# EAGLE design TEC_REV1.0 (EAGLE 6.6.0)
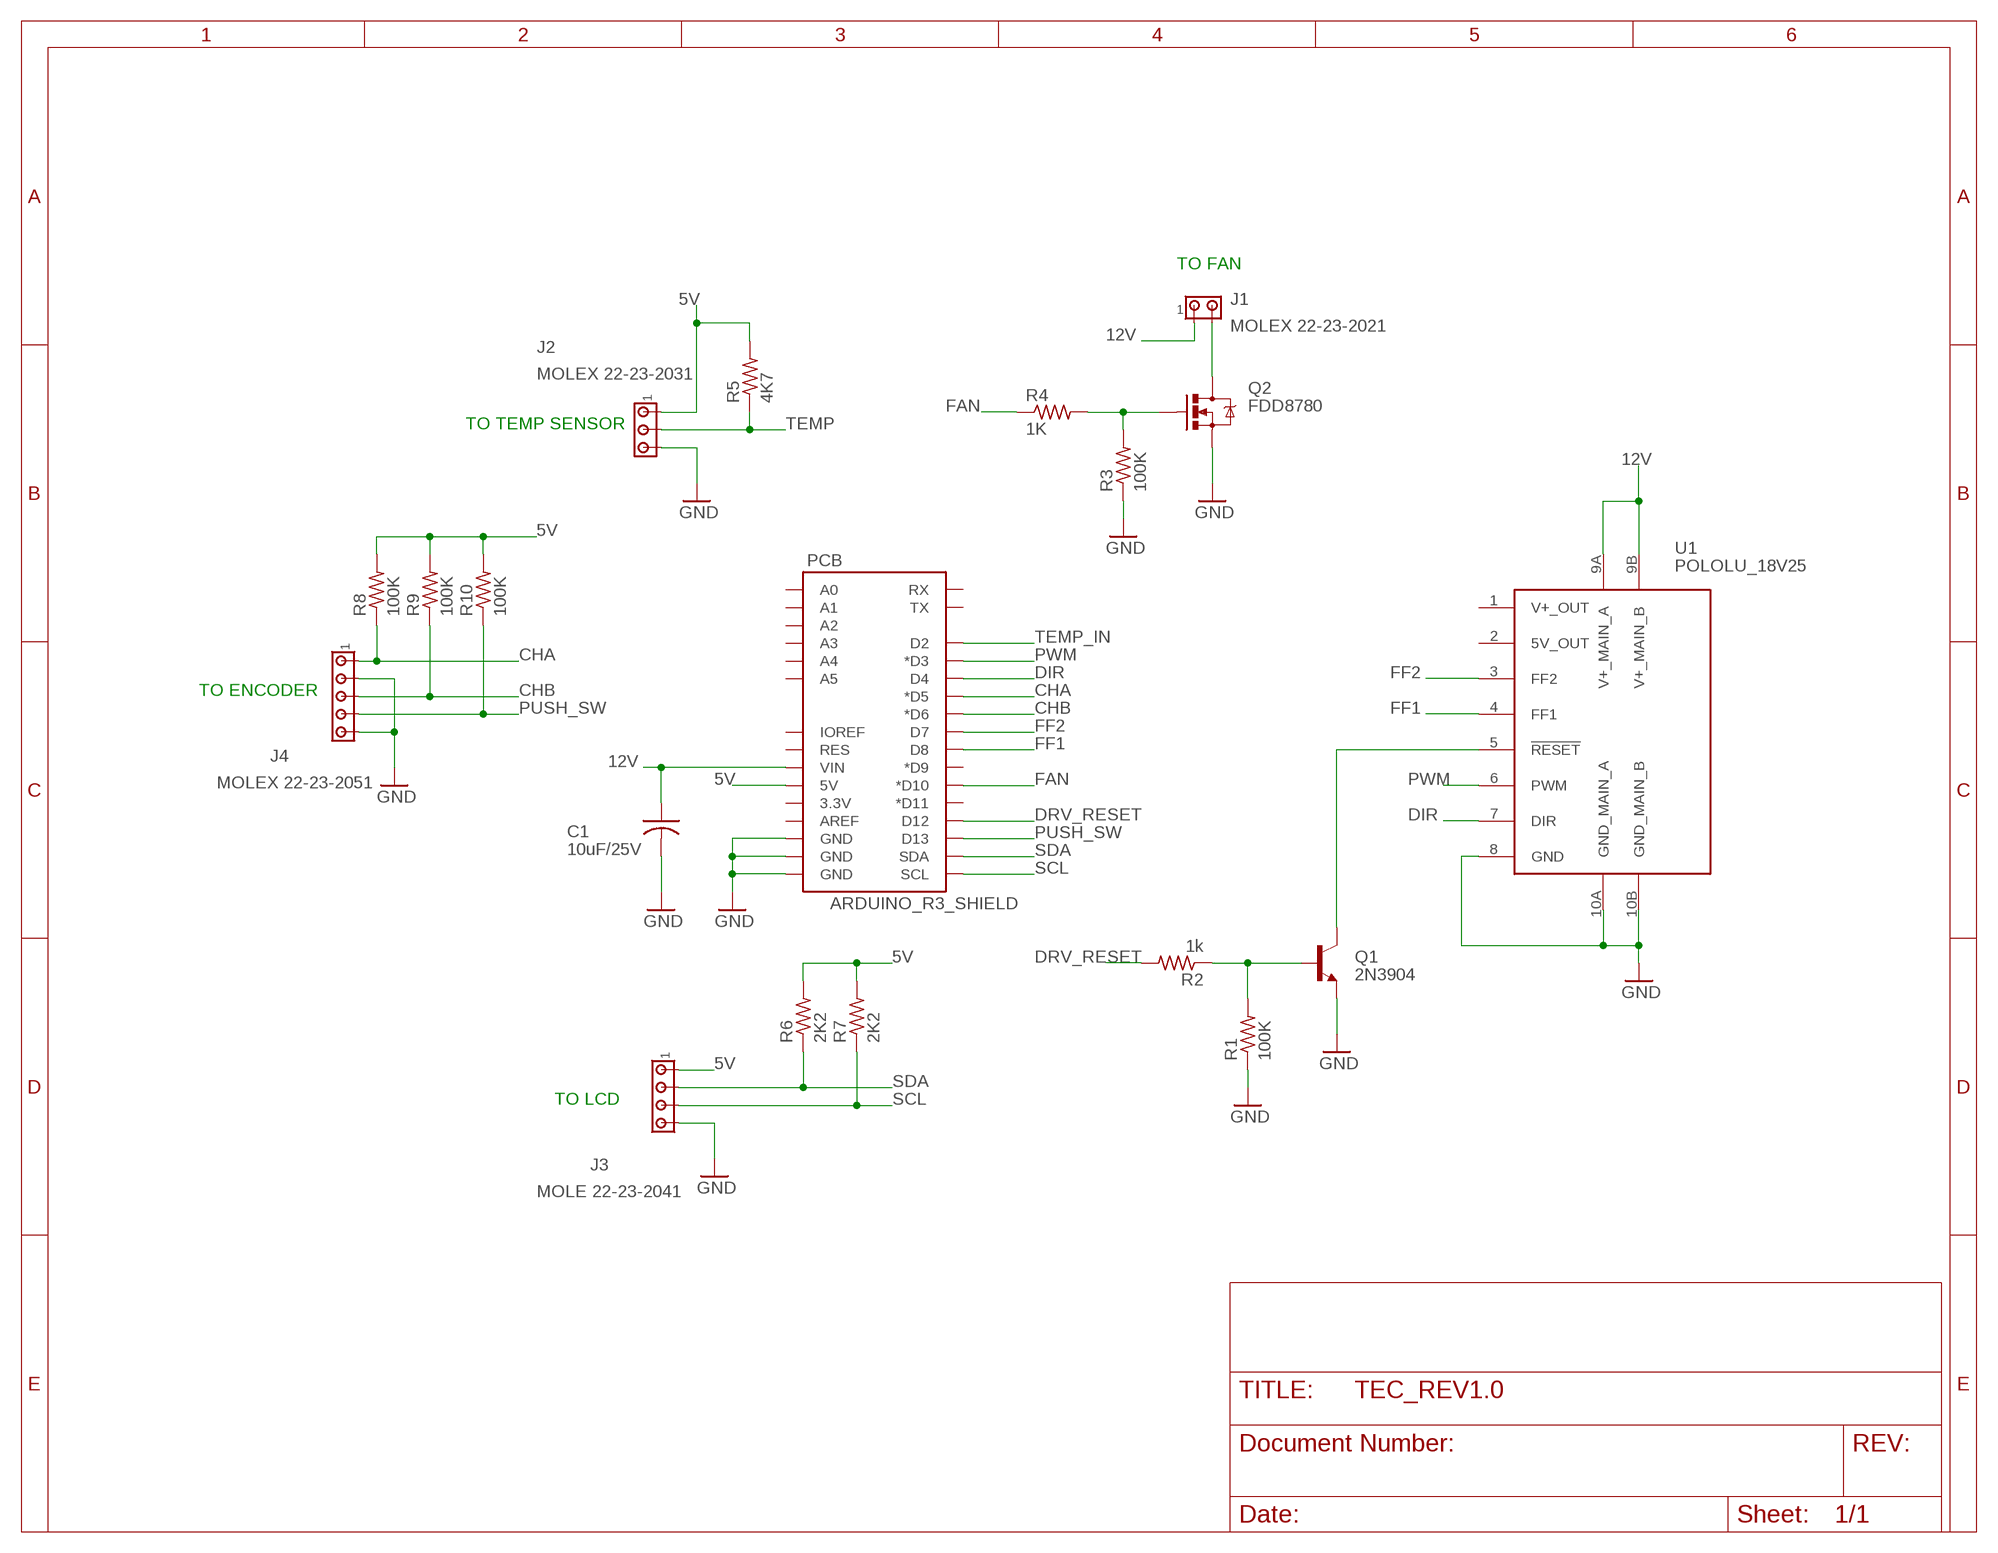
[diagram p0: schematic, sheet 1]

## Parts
C1  10uF/25V  C-USC0603  [C0603]
J1  MOLEX 22-23-2021  MTA02-100  [10X02MTA]
J2  MOLEX 22-23-2031  MTA03-100  [10X03MTA]
J3  MOLE 22-23-2041  MTA04-100  [10X04MTA]
J4  MOLEX 22-23-2051  MTA05-100  [10X05MTA]
PCB  ARDUINO_R3_SHIELD  [UNO_R3_SHIELD]
Q1  2N3904  TRANSISTOR_NPNSOT23  [SOT23]
Q2  FDD8780  MOSFET-NCHANNELFDD8780  [DPAK]
R1  100K  R-US_R0603  [R0603]
R2  1k  R-US_R0603  [R0603]
R3  100K  R-US_R0603  [R0603]
R4  1K  R-US_R0603  [R0603]
R5  4K7  R-US_R0603  [R0603]
R6  2K2  R-US_R0603  [R0603]
R7  2K2  R-US_R0603  [R0603]
R8  100K  R-US_R0603  [R0603]
R9  100K  R-US_R0603  [R0603]
R10  100K  R-US_R0603  [R0603]
U1  POLOLU_18V25  [POLOLU_18V25]

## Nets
5V: J2.1 J3.1 PCB.5V R5.2 R6.2 R7.2 R8.2 R9.2 R10.2
12V: C1.1 J1.1 PCB.VIN U1.9A(V+_MAIN_A) U1.9B(V+_MAIN_B)
CHA: J4.1 PCB.D5(*D5) R8.1
CHB: J4.3 PCB.D6(*D6) R9.1
DIR: PCB.D4 U1.7(DIR)
DRV_RESET: PCB.D12 R2.2
FAN: PCB.D10(*D10) R4.1
FF1: PCB.D8 U1.4(FF1)
FF2: PCB.D7 U1.3(FF2)
GND: C1.2 J2.3 J3.4 J4.2 J4.5 PCB.GND@0(GND) PCB.GND@1(GND) PCB.GND@2(GND) Q1.2(E) Q2.3(S) R1.1 R3.1 U1.8(GND) U1.10A(GND_MAIN_A) U1.10B(GND_MAIN_B)
N$2: Q1.3(C) U1.5(!RESET)
N$3: J1.2 Q2.4(D)
N$5: Q2.1(G) R3.2 R4.2
N$6: Q1.1(B) R1.2 R2.1
PUSH_SW: J4.4 PCB.D13 R10.1
PWM: PCB.D3(*D3) U1.6(PWM)
SCL: J3.3 PCB.SCL R7.1
SDA: J3.2 PCB.SDA R6.1
TEMP: J2.2 R5.1
TEMP_IN: PCB.D2
Unconnected: PCB.3.3V PCB.A0 PCB.A1 PCB.A2 PCB.A3 PCB.A4 PCB.A5 PCB.AREF PCB.D9(*D9) PCB.D11(*D11) PCB.IOREF PCB.RES PCB.RX PCB.TX U1.1(V+_OUT) U1.2(5V_OUT)

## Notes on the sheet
- TO FAN
- TO TEMP SENSOR
- TO ENCODER
- TO LCD

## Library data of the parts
C1 = rcl:C-US: CAPACITOR, American symbol
J1 = con-amp:MTA02-100: AMP connector
J2 = con-amp:MTA03-100: AMP connector
J3 = con-amp:MTA04-100: AMP connector
J4 = con-amp:MTA05-100: AMP connector
PCB = SparkFun-Boards:ARDUINO_R3_SHIELD: Shield form compatible with the Arduino Uno R3.
Q1 = SparkFun-DiscreteSemi:TRANSISTOR_NPN: Generic NPN BJT MMBT2222A - TRANS-08049 (SOT-23, 1A 40V) MPSA42 - TRANS-09116 (SOT-23, 500mA 300V) MMBT5088LT1G - TRANS-11160 (SOT-23, 50 mA 30V)
Q2 = SparkFun-DiscreteSemi:MOSFET-NCHANNEL: Common NMOSFET Parts MFG P/NStore IDProd ID FDD8780TRANS-09984 SI7820DNTRANS-11055 FDS6630AIC-08089 2N7002PWTRANS-11151 FQP30N06L COM-10213TRANS-10060 BSS123LT1GTRANS-08345 BSS138TRANS-00830 BS170 2N7000; PROD_ID: TRANS-09984
R1-R10 = rcl:R-US_: RESISTOR, American symbol
U1 = Dartronix:POLOLU_18V25

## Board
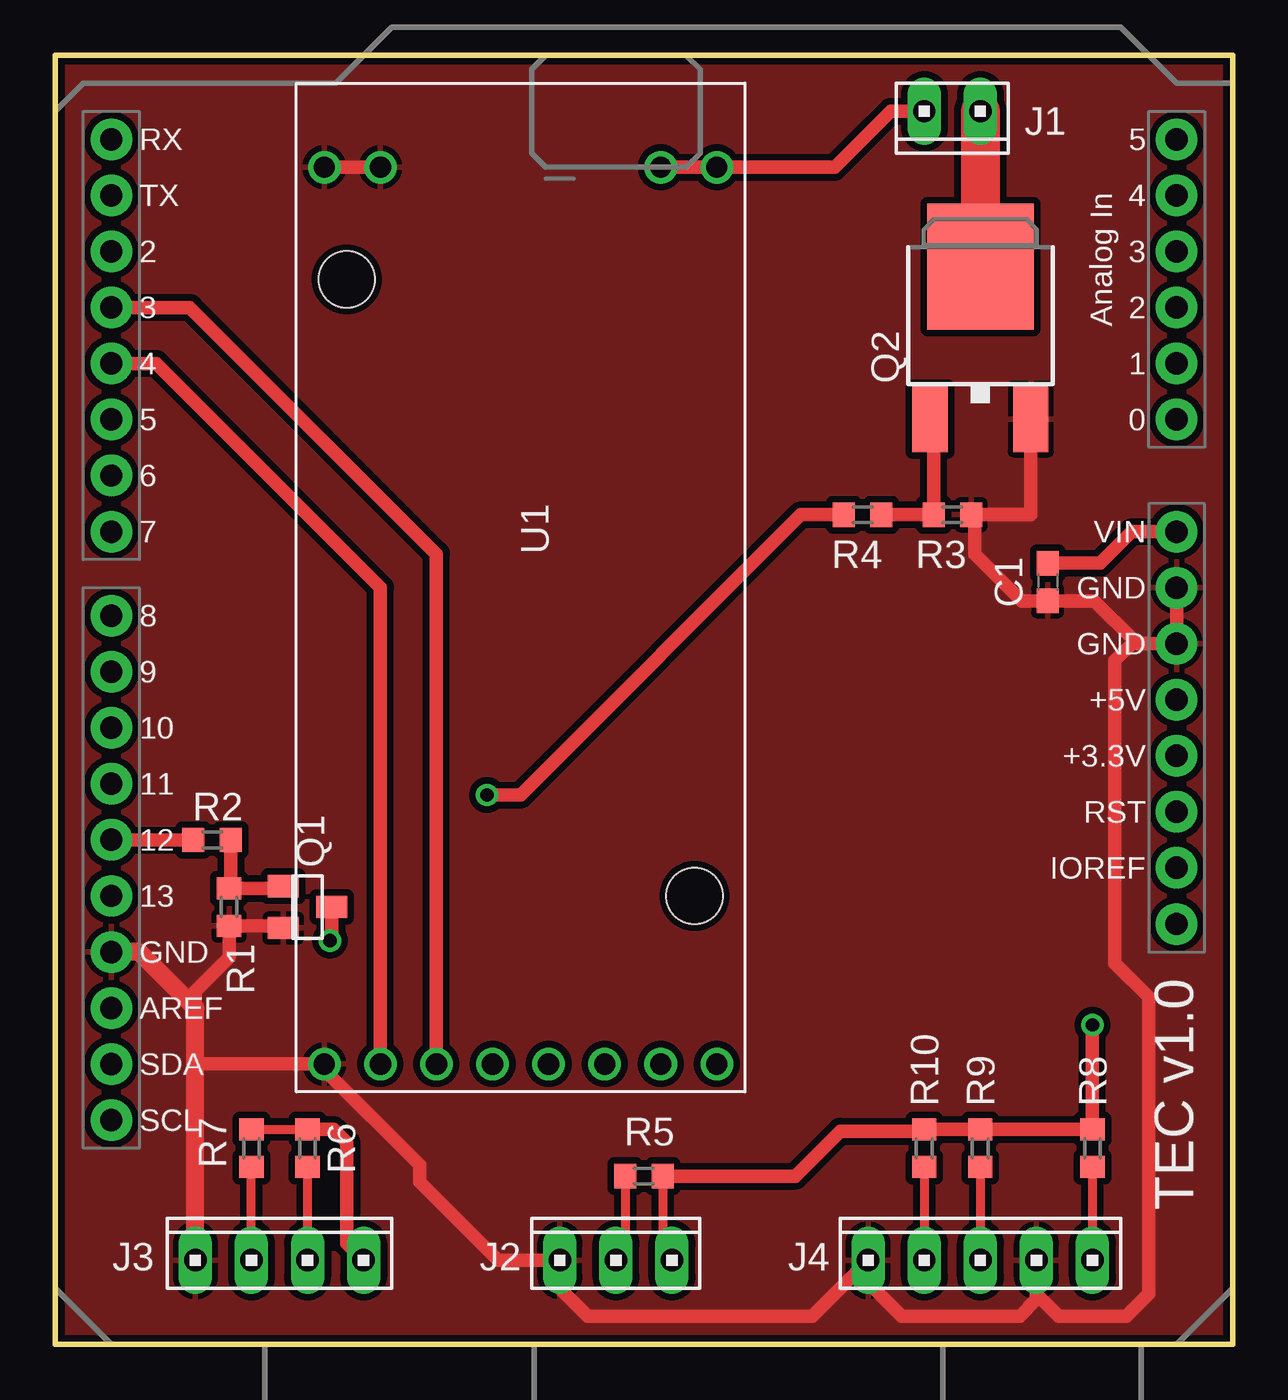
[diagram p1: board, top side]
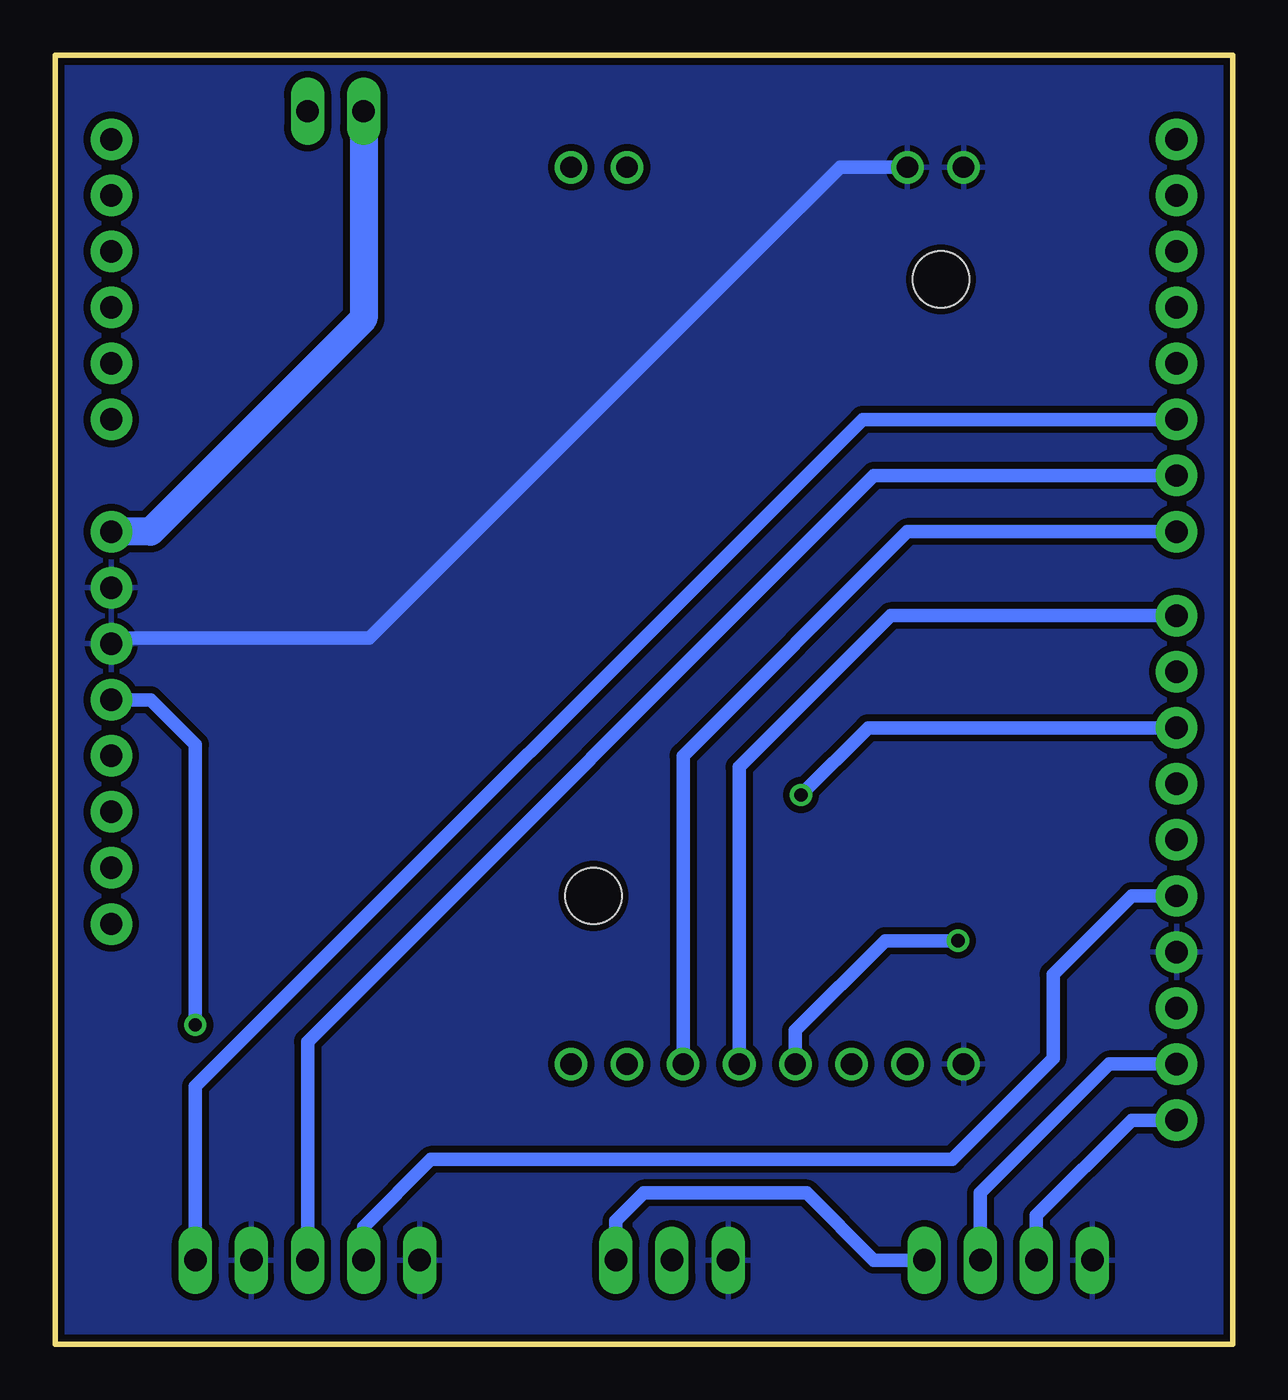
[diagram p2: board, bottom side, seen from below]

Size 53.34 x 58.42 mm. Coordinates in mm from the lower left corner, seen from the top.
Outline: 0,0 53.34,0 53.34,58.42 0,58.42 0,0
Copper layers (1*16): Top 0.035mm / dielectric 1.5mm / Bottom 0.035mm
Design rules "default *": minimum track width 10mil, minimum drill 24mil, track to track 8mil, track to pad 8mil, pad to pad 8mil, via to via 8mil, smd to smd 8mil, copper to edge 10mil, drill to drill 8mil, minimum pad ring 10mil, minimum via ring 8mil, stop-mask expansion 4mil, vias tented up to drill 0mil, thermal gap 10mil

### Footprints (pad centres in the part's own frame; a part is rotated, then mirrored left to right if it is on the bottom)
C0603 = smd 1.1 x 1: 1 -0.85,0; 2 0.85,0
10X02MTA = drill 1.016 long: 1 1.27,0; 2 -1.27,0
10X03MTA = drill 1.016 long: 1 2.54,0; 2 0,0; 3 -2.54,0
10X04MTA = drill 1.016 long: 1 3.81,0; 2 1.27,0; 3 -1.27,0; 4 -3.81,0
10X05MTA = drill 1.016 long: 1 5.08,0; 2 2.54,0; 3 0,0; 4 -2.54,0; 5 -5.08,0
UNO_R3_SHIELD = drill 1.016 pad 1.88: 3.3V 50.8,26.67; 5V 50.8,29.21; A0 50.8,41.91; A1 50.8,44.45; A2 50.8,46.99; A3 50.8,49.53; A4 50.8,52.07; A5 50.8,54.61; AREF 2.54,15.24; D2 2.54,49.53; D3 2.54,46.99; D4 2.54,44.45; D5 2.54,41.91; D6 2.54,39.37; D7 2.54,36.83; D8 2.54,33.02; D9 2.54,30.48; D10 2.54,27.94; D11 2.54,25.4; D12 2.54,22.86; D13 2.54,20.32; GND@0 50.8,31.75; GND@1 50.8,34.29; GND@2 2.54,17.78; IOREF 50.8,21.59; NC 50.8,19.05; RES 50.8,24.13; RX 2.54,54.61; SCL 2.54,10.16; SDA 2.54,12.7; TX 2.54,52.07; VIN 50.8,36.83
SOT23 = smd 1 x 1.4: 1 -0.95,-1.1; 2 0.95,-1.1; 3 0,1.1
DPAK = smd 1.6 x 3: 1 -2.28,-5.31; 3 2.28,-5.31 | smd 4.826 x 5.715: 4 0,1.588
R0603 = smd 1 x 1.1: 1 -0.85,0; 2 0.85,0
POLOLU_18V25 = drill 0.965: 1 44.45,19.05; 2 44.45,16.51; 3 44.45,13.97; 4 44.45,11.43; 5 44.45,8.89; 6 44.45,6.35; 7 44.45,3.81; 8 44.45,1.27; 9A 3.81,19.05; 9B 3.81,16.51; 10A 3.81,3.81; 10B 3.81,1.27 | hole 2.54: 36.83,18.034; 8.89,2.286

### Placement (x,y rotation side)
C1  44.96,34.54 270 top
J1  40.64,55.88 180 top
J2  25.4,3.81 0 top
J3  10.16,3.81 0 top
J4  41.91,3.81 0 top
PCB  0,0 0 top
Q1  11.43,19.81 270 top
Q2  41.91,47.24 0 top
R1  7.87,19.81 90 top
R2  7.11,22.86 180 top
R3  40.64,37.59 180 top
R4  36.58,37.59 0 top
R5  26.67,7.62 0 top
R6  11.43,8.89 90 top
R7  8.89,8.89 90 top
R8  46.99,8.89 90 top
R9  41.91,8.89 90 top
R10  39.37,8.89 90 top
U1  10.92,57.15 270 top

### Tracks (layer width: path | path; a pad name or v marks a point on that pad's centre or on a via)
5V  (via drill 0.6)
  Top 0.406: R7.2 R6.2 | R5.2 27.52,4.23 J2.1
  Top 0.61: R5.2 33.53,7.62 35.56,9.65 39.28,9.65 R10.2 R9.2 R8.2 v46.99,14.48 | R6.2 12.61,9.74 13.21,9.14 13.21,4.57 J3.1
  Bottom 0.61: J3.1 16.26,3.81 19.3,6.86 26.67,6.86 27.94,5.59 J2.1 | v46.99,14.48 46.99,27.18 49.02,29.21 PCB.5V
12V
  Top 0.61: C1.1 47.33,35.39 48.77,36.83 PCB.VIN | U1.9B U1.9A 35.31,53.34 37.85,55.88 J1.1
  Bottom 1.27: J1.1 39.37,46.48 49.02,36.83 PCB.VIN
CHA
  Top 0.406: R8.1 J4.1
  Bottom 0.61: PCB.D5 16.76,41.91 46.99,11.68 J4.1
CHB
  Top 0.406: R9.1 J4.3
  Bottom 0.61: PCB.D6 16.26,39.37 41.91,13.72 J4.3
DIR
  Top 0.61: U1.7 14.73,34.29 4.57,44.45 PCB.D4
DRV_RESET
  Top 0.61: PCB.D12 R2.2
FAN  (via drill 0.6)
  Top 0.61: v19.56,24.89 21.08,24.89 33.78,37.59 R4.1
  Bottom 0.61: PCB.D10 16.51,27.94 v19.56,24.89
FF1
  Bottom 0.61: PCB.D8 15.49,33.02 22.35,26.16 U1.4
FF2
  Bottom 0.61: PCB.D7 14.73,36.83 24.89,26.67 U1.3
GND
  Top 0.61: Q1.2 10.23,18.96 R1.1 7.87,17.53 6.35,16 6.35,15.24 | 6.35,12.7 U1.8 12.19,12.45 16.51,8.13 16.51,7.37 20.07,3.81 J2.3 22.86,2.54 24.13,1.27 34.29,1.27 J4.5 36.83,2.79 38.35,1.27 43.69,1.27 44.45,2.03 J4.2 44.45,2.29 45.47,1.27 48.51,1.27 49.53,2.29 49.53,15.75 48.01,17.27 48.01,30.99 48.9,31.88 | PCB.GND@1 PCB.GND@0 49.02,31.75 48.9,31.88 | 48.9,31.88 47.08,33.69 C1.2 43.78,33.69 41.66,35.81 41.66,37.43 R3.1 44.2,37.59 Q2.3 | U1.10B U1.10A
  Top 0.813: J3.4 6.35,12.7 6.35,15.24 3.81,17.78 PCB.GND@2
  Bottom 0.61: U1.10A 17.78,53.34 39.12,32 50.55,32 PCB.GND@0
  pour Bottom (isolate 0.305): 0.25,58.17 53.09,58.17 53.09,0.25 0.25,0.25
  pour Top (isolate 0.305): 0.25,58.17 53.09,58.17 53.09,0.25 0.25,0.25
N$2  (via drill 0.6)
  Top 0.61: Q1.3 12.53,18.37 v12.45,18.29
  Bottom 0.61: v12.45,18.29 15.75,18.29 19.81,14.22 U1.5
N$3
  Top 1.778: J1.2 Q2.4
N$5
  Top 0.61: R4.2 R3.2 39.79,41.77 Q2.1
N$6
  Top 0.61: R2.1 7.96,20.75 R1.2 10.23,20.66 Q1.1
PUSH_SW
  Top 0.406: R10.1 J4.4
  Bottom 0.61: PCB.D13 4.57,20.32 8.13,16.76 8.13,12.95 12.7,8.38 36.32,8.38 39.37,5.33 J4.4
PWM
  Top 0.61: U1.6 17.27,35.81 6.1,46.99 PCB.D3
SCL
  Top 0.406: J3.3 R7.1
  Bottom 0.61: PCB.SCL 4.57,10.16 8.89,5.84 J3.3
SDA
  Top 0.406: J3.2 R6.1
  Bottom 0.61: PCB.SDA 5.59,12.7 11.43,6.86 J3.2
TEMP
  Top 0.406: R5.1 25.82,4.23 J2.2

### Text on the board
tPlace: TEC v1.0

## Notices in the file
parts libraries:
SparkFun-Boards: Licensing: CC v3.0 Share-Alike You are welcome to use this library for commercial purposes.
